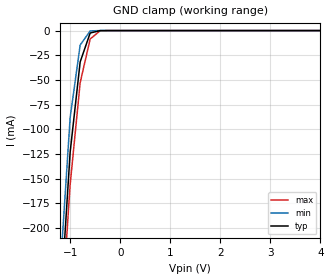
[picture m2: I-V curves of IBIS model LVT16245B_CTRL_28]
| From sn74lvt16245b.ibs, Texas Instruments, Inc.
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|  Model LVT16245B Input CTRL_28
[Model]   LVT16245B_CTRL_28
Model_type  Input
Polarity   Inverting
Vinl = 0.8V
Vinh = 2.0V
| variable   typ   min   max
C_comp   4p   NA   NA
[Temperature Range]   40   -25   100
| Ambient Temperature   25   -40   85
[Voltage range]   2.8   2.7   2.9
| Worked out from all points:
|   GND clamp passes 1 mA (typ) near -0.48 V on its own axis
[GND Clamp]
|   Voltage   I(typ)   I(min)   I(max)
-5V       -4.255A    -4.666A    -3.859A
-1.2V     -283.6mA   -244.5mA   -309.8mA
-1V       -123mA     -88.01mA   -155.8mA
-800mV    -31.69mA   -14.66mA   -52.76mA
-600mV    -2.458mA   -341.6uA   -8.418mA
-400mV    -7.655uA   -383.7nA   -219.5uA
5V        259.3pA    2.847uA    716.5pA
